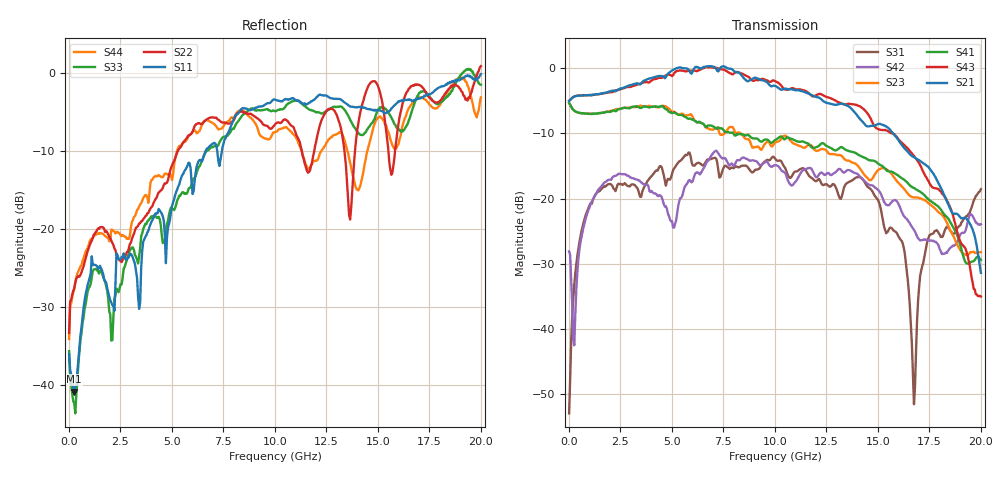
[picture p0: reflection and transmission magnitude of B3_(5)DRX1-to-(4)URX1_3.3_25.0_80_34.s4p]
!Agilent Technologies,N5225A,MY51451112,A.09.50.13
!Agilent N5225A: A.09.50.13
!Date: Sunday, March 12, 2017 05:21:02
!Correction: S11(Full 4 Port(1,2,3,4))
!S12(Full 4 Port(1,2,3,4))
!S13(Full 4 Port(1,2,3,4))
!S14(Full 4 Port(1,2,3,4))
!S21(Full 4 Port(1,2,3,4))
!S22(Full 4 Port(1,2,3,4))
!S23(Full 4 Port(1,2,3,4))
!S24(Full 4 Port(1,2,3,4))
!S31(Full 4 Port(1,2,3,4))
!S32(Full 4 Port(1,2,3,4))
!S33(Full 4 Port(1,2,3,4))
!S34(Full 4 Port(1,2,3,4))
!S41(Full 4 Port(1,2,3,4))
!S42(Full 4 Port(1,2,3,4))
!S43(Full 4 Port(1,2,3,4))
!S44(Full 4 Port(1,2,3,4))
!S4P File: Measurements: <S11,S12,S13,S14>,
!<S21,S22,S23,S24>,
!<S31,S32,S33,S34>,
!<S41,S42,S43,S44>:
# Hz S  dB  R 50
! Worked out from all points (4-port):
!   401 points, 10 MHz to 20 GHz, reference 50 ohm
!   strongest paths, dB at 10 MHz, 5.008 GHz, 10.01 GHz, 15 GHz, 20 GHz:
!     S21: -5.0, -0.4, -2.7, -8.6, -31.4
!     S43: -5.0, -1.2, -2.0, -9.3, -35.0
!     S41: -5.3, -6.9, -11.0, -14.6, -29.4
!     S23: -5.3, -6.7, -11.4, -15.7, -28.2
!     S42: -28.1, -23.5, -14.9, -18.6, -23.9
!     S31: -52.9, -16.2, -13.8, -20.2, -18.6
!   lowest |S11| = -40.9 dB at 259.9 MHz (marker M1), VSWR 1.02, Z = 50.3 - j0.866 ohm
!   |S11| at or under -10 dB: start of sweep to 6.645 GHz; 7.197 GHz to 7.43 GHz (232.8 MHz wide, 3.18 % of centre)
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1e7  -36.11 -39.6  -63.24 139.7  -52.94 22.4  -66.88 145.5
     -5.02 1.3  -33.37 39.3  -5.33 179.9  -28.01 38.0
     -52.92 11.3  -64.30 138.8  -35.72 -46.0  -71.75 127.6
     -5.34 179.9  -28.09 38.0  -5.00 1.5  -34.17 44.2
2.59875e8  -40.90 -72.7  -49.79 57.4  -33.14 95.0  -50.58 52.6
           -4.36 -5.7  -27.65 -131.6  -6.52 165.1  -42.06 -161.8
           -33.22 95.2  -50.08 57.5  -42.39 -79.1  -50.77 56.4
           -6.52 164.3  -42.51 -170.5  -4.35 -6.5  -27.70 -137.7
5.2074e9  -15.29 86.0  -35.95 10.7  -15.02 30.1  -37.52 -4.7
          -0.03 174.6  -10.61 142.4  -6.95 -35.2  -23.67 65.4
          -14.89 28.3  -36.31 8.2  -16.90 102.7  -42.61 -22.0
          -6.92 -51.5  -23.30 65.1  -0.49 164.6  -10.51 120.5
8.30585e9  -4.86 37.8  -39.48 -99.9  -15.20 -1.8  -36.57 -139.7
           -0.82 24.0  -4.98 79.6  -9.91 -151.8  -13.83 47.3
           -15.12 -2.2  -32.61 -123.8  -5.88 57.7  -32.04 -161.6
           -10.09 -174.7  -14.11 50.3  -0.73 11.3  -4.83 44.8
1.225388e10  -2.89 -19.7  -34.81 -160.9  -17.41 -23.7  -36.37 160.2
             -4.78 -141.2  -6.15 71.1  -12.41 53.7  -15.93 37.7
             -17.67 -22.5  -34.40 -149.1  -5.24 -7.3  -33.39 164.8
             -11.56 15.3  -16.00 40.3  -4.01 -166.8  -10.06 -6.2
1.68016e10  -3.50 -76.5  -35.63 110.9  -55.52 -126.2  -36.41 82.9
            -13.73 23.0  -1.50 70.2  -19.82 -177.7  -25.25 62.6
            -48.82 -154.4  -32.93 122.9  -3.71 -82.9  -33.47 81.2
            -18.47 130.7  -25.08 62.8  -13.72 -29.4  -3.50 -60.5
2e10  -0.18 -114.1  -33.00 63.0  -18.60 121.7  -35.49 21.2
      -31.38 -120.5  0.84 17.1  -28.21 45.3  -23.90 102.0
      -18.57 121.7  -34.01 40.1  -1.54 -87.6  -35.30 -8.2
      -29.40 4.3  -23.93 102.7  -35.01 -146.0  -3.17 -136.5
